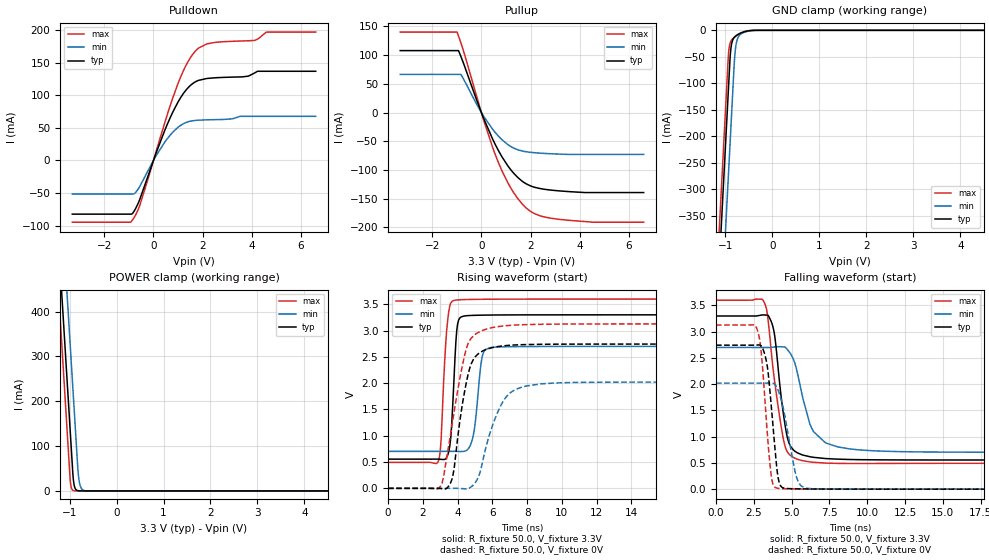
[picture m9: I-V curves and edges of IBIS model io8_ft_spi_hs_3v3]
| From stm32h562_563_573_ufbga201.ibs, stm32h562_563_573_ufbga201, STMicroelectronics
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[Model]   io8_ft_spi_hs_3v3
Model_type I/O
Polarity   Non-Inverting
Enable   Active-Low
| CAP_THRESHOLD on pad IOFT is "UDTCAPC" :
| Rising=20.0% of vddiom   Falling=80.0% of vddiom
| C_comp min and max val. don't necessarily correlate with the min and max pvt
| but are the smallest and greatest pad capacitance found.
| var   typ   min   max
C_comp   5.03687pF  4.97376pF  5.04455pF
|C_comp_pullup   3.26810pF  3.10735pF  3.04315pF
|C_comp_pulldown   1.76877pF  1.86641pF  2.00140pF
Vinl = 810.0mV
Vinh = 2.52V
Vmeas = 1.65V   | Reference voltage for timing measurements
Cref  = 50.0pF   | Timing specification test load capacitance value
Rref  = 100.0MOhm   | Timing specification test load resistance value
Vref  = 1.65V   | Timing specification test load voltage
[Model Spec]
| TIME_THRESHOLD on pin ZIV11 is "CMOS" :
| Rising=40.0% of vdd   Falling=60.0% of vdd
Vinl 1.29880V 1.07480V 1.40680V
Vinh 1.77520V 1.49320V 1.89720V
| variable   typ   min   max
[Temperature Range] 25.0 125.0 -40.0
| variable   typ   min   max
[Voltage Range] 3.3V 2.7V 3.6V
| variable   typ   min   max
[POWER Clamp Reference] 3.3V 2.7V 3.6V
| variable   typ   min   max
[GND Clamp Reference] 0V 0V 0V
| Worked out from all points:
|   slope of the pulldown table from 0 to 0.495 V, typ, clamps not added: 10 ohm
|   slope of the pullup table from 0 to 0.495 V, typ, clamps not added: 10 ohm
|   GND clamp passes 1 mA (typ) near -0.52 V on its own axis
|   POWER clamp passes 1 mA (typ) near -0.84 V on its own axis
|   rising waveform, R_fixture 50.0, V_fixture 3.3V: 20-80 % time 257ps typ, 366ps min, 290ps max; typ from 0.556 V to 3.3 V
|   falling waveform, R_fixture 50.0, V_fixture 3.3V: 20-80 % time 681ps typ, 1.13ns min, 820ps max; typ from 3.3 V to 0.556 V
|   rising waveform, R_fixture 50.0, V_fixture 0V: 20-80 % time 765ps typ, 1.18ns min, 991ps max; typ from 0 V to 2.74 V
|   falling waveform, R_fixture 50.0, V_fixture 0V: 20-80 % time 515ps typ, 790ps min, 494ps max; typ from 2.74 V to 0 V
[POWER Clamp]
-3.3V     4.068A     4.259A     3.957A
-1.25V    582.8mA    774.2mA    471.5mA
-1.13V    378.8mA    570.2mA    267.5mA
-1.09V    310.8mA    502.2mA    199.5mA
-1.02V    191.8mA    383.2mA    80.53mA
-990mV    140.8mA    332.2mA    29.53mA
-920mV    26.3mA     213.2mA    906uA
-880mV    5.543mA    145.2mA    123.7uA
-810mV    363.5uA    33.6mA     3.798uA
-770mV    76.62uA    10.47mA    519.4nA
-690mV    3.409uA    1.017mA    10.48nA
6.6V      0A         0A         0A
[GND Clamp]
-3.3V     -4.131A    -4.293A    -4.064A
-1.25V    -646.2mA   -808mA     -579.5mA
-940mV    -119.2mA   -281mA     -52.48mA
-920mV    -85.23mA   -247mA     -32.7mA
-900mV    -51.91mA   -213mA     -24.27mA
-870mV    -26.87mA   -162mA     -18.7mA
-810mV    -13.22mA   -60.41mA   -13.31mA
-790mV    -11.41mA   -38.37mA   -11.93mA
-740mV    -8.18mA    -15.37mA   -8.882mA
-660mV    -4.605mA   -6.274mA   -4.919mA
-320mV    -10.56uA   -77.76uA   -2.038uA
6.6V      9.514nA    1.879uA    704.5pA
| variable   typ   min   max
[Pullup Reference] 3.3V 2.7V 3.6V
| variable   typ   min   max
[Pulldown Reference] 0V 0V 0V
[Pullup]
-3.3V     107.8mA    66.41mA    140mA
-990mV    107.8mA    66.41mA    140mA
-930mV    107.8mA    66.41mA    133.1mA
-830mV    97.2mA     66.41mA    120.9mA
120mV     -12.96mA   -8.365mA   -16.99mA
680mV     -65.11mA   -40.43mA   -85.66mA
1.26V     -102.9mA   -60.65mA   -135.8mA
1.85V     -124.7mA   -68.43mA   -167.2mA
2.35V     -132mA     -70.55mA   -179.2mA
3.24V     -136.6mA   -72.47mA   -186.2mA
4.54V     -139.3mA   -72.9mA    -190.8mA
6.6V      -139.3mA   -72.9mA    -190.8mA
[Pulldown]
-3.3V     -82.43mA   -51.49mA   -94.82mA
-860mV    -81.66mA   -51.49mA   -91.78mA
-560mV    -60.16mA   -40.13mA   -69.41mA
120mV     12.61mA    7.999mA    15.37mA
800mV     75.3mA     43.94mA    97.52mA
1.33V     108.3mA    58.37mA    146.5mA
1.84V     123.1mA    61.83mA    172.7mA
2.51V     126.9mA    62.7mA     181.3mA
3.84V     129.3mA    67.77mA    183.7mA
4.13V     134.7mA    67.77mA    184.6mA
4.59V     136.9mA    67.77mA    197.1mA
6.6V      136.9mA    67.77mA    197.1mA
[Ramp]
dV/dt_r 1.64628V/761.24141ps 1.21235V/1.18056ns 1.87635V/990.019ps
dV/dt_f 1.64666V/679.90796ps 1.19801V/1.12358ns 1.86387V/819.73862ps
R_load = 50.0
| Removed startup time: 0s 0s 0s  .
| Removed end time: 19.4ns.
[Rising Waveform]
R_fixture   = 50.0
V_fixture   = 3.3V
V_fixture_min = 2.7V
V_fixture_max = 3.6V
0s        555.6mV    703.3mV    493.6mV
2.9ns     555.2mV    703.3mV    527.3mV
3.05ns    551.4mV    703.3mV    928.7mV
3.4ns     606.6mV    703.3mV    3.104V
3.6ns     941.8mV    703.3mV    3.519V
3.75ns    1.79V      703.3mV    3.569V
4.05ns    3.193V     700.9mV    3.585V
4.85ns    3.289V     935.3mV    3.594V
5.6ns     3.295V     2.64V      3.596V
19.4ns    3.3V       2.7V       3.6V
| Removed startup time: 0s 0s 0s  .
| Removed end time: 39.4ns.
[Falling Waveform]
R_fixture   = 50.0
V_fixture   = 3.3V
V_fixture_min = 2.7V
V_fixture_max = 3.6V
0s        3.3V       2.7V       3.6V
3.15ns    3.32V      2.7V       3.582V
3.4ns     3.318V     2.699V     3.327V
3.8ns     3.052V     2.706V     2.231V
4.5ns     1.347V     2.712V     893.4mV
4.9ns     831.9mV    2.593V     648.1mV
5.65ns    659mV      1.856V     547.7mV
6.45ns    606.7mV    1.095V     511.8mV
8.85ns    565.3mV    766.6mV    489.2mV
39.4ns    555.6mV    703.3mV    493.6mV
| Removed startup time: 0s 0s 0s  .
| Removed end time: 39.3ns.
[Rising Waveform]
R_fixture   = 50.0
V_fixture   = 0V
V_fixture_min = 0V
V_fixture_max = 0V
0s        103.7nV    446.4nV    93.92nV
2.9ns     -7.525uV   1.759uV    -1.085mV
3.5ns     49.02mV    72.25uV    842.1mV
3.8ns     373.9mV    305.7uV    1.456V
4.7ns     2.288V     10.63mV    2.816V
5.2ns     2.562V     220.1mV    2.967V
5.9ns     2.669V     1.091V     3.05V
6.9ns     2.718V     1.778V     3.097V
8.8ns     2.74V      1.987V     3.12V
39.3ns    2.744V     2.021V     3.127V
| Removed startup time: 0s 0s 0s  .
| Removed end time: 19.4ns.
[Falling Waveform]
R_fixture   = 50.0
V_fixture   = 0V
V_fixture_min = 0V
V_fixture_max = 0V
0s        2.744V     2.021V     3.127V
2.7ns     2.746V     2.021V     3.059V
3ns       2.725V     2.021V     2.577V
3.4ns     2.324V     2.023V     1.036V
3.7ns     1.433V     2.024V     172.8mV
3.95ns    611.8mV    1.976V     29.32mV
4.3ns     52.69mV    1.713V     11.1mV
5.3ns     6.425mV    254mV      4.259mV
5.95ns    4.24mV     17.5mV     2.874mV
19.4ns    8.738uV    39.37uV    9.334uV
